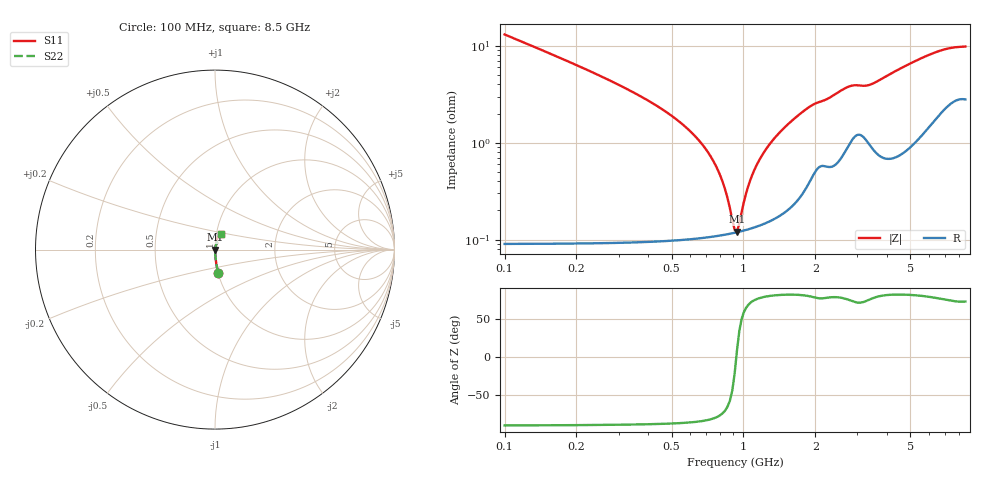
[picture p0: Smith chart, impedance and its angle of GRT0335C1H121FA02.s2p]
!Murata Part Number: GRT0335C1H121FA02
!These Parameters are Measured in Series Mode Connection
!Data Generated on Jun 19, 2026
!  o--ll--o
!Port1  Port2
!  o------o
!Operation Temp=25[degC], DC Bias Voltage=0[V]
!Freq. Start=100[MHz] Stop=9[GHz] 401[Steps]
# Hz S RI R 50
!Freq.(Hz) S11(Real) S11(Imag) S21(Real) S21(Imag) S12(Real) S12(Imag) S22(Real) S22(Imag)
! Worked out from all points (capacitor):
!   401 points, 100 MHz to 8.5 GHz, reference 50 ohm
!   read as one part in series: C = 120 pF near 142 MHz
!   lowest |Z| = 121 mohm at 940 MHz (marker M1)
!   series resonance near 933.6 MHz, so ESL is about 240 pH
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1e8  0.0178 -0.1287  0.9822 0.1287  0.9822 0.1287  0.0178 -0.1287
2.05e8  0.00468 -0.0613  0.9953 0.0613  0.9953 0.0613  0.00468 -0.0613
2.68e8  0.00298 -0.0453  0.997 0.0453  0.997 0.0453  0.00298 -0.0453
5.83e8  0.0012 -0.0139  0.9988 0.0139  0.9988 0.0139  0.0012 -0.0139
7.09e8  0.00112 -0.00796  0.9989 0.00796  0.9989 0.00796  0.00112 -0.00796
8.14e8  0.00113 -0.00393  0.9989 0.00393  0.9989 0.00393  0.00113 -0.00393
8.98e8  0.00116 -0.00111  0.9988 0.00111  0.9988 0.00111  0.00116 -0.00111
9.19e8  0.00118 -0.000451  0.9988 0.000451  0.9988 0.000451  0.00118 -0.000451
9.4e8  0.00119 0.000197  0.9988 -0.000197  0.9988 -0.000197  0.00119 0.000197
9.61e8  0.00121 0.000832  0.9988 -0.000832  0.9988 -0.000832  0.00121 0.000832
1.066e9  0.00131 0.00384  0.9987 -0.00384  0.9987 -0.00384  0.00131 0.00384
1.15e9  0.00141 0.00607  0.9986 -0.00607  0.9986 -0.00607  0.00141 0.00607
1.297e9  0.00165 0.00974  0.9984 -0.00974  0.9984 -0.00974  0.00165 0.00974
1.507e9  0.00216 0.0147  0.9978 -0.0147  0.9978 -0.0147  0.00216 0.0147
1.948e9  0.00505 0.0239  0.9949 -0.0239  0.9949 -0.0239  0.00505 0.0239
2.662e9  0.00921 0.035  0.9908 -0.035  0.9908 -0.035  0.00921 0.035
2.914e9  0.0127 0.0366  0.9873 -0.0366  0.9873 -0.0366  0.0127 0.0366
3.376e9  0.0108 0.0377  0.9892 -0.0377  0.9892 -0.0377  0.0108 0.0377
4.3e9  0.00979 0.053  0.9902 -0.053  0.9902 -0.053  0.00979 0.053
5.707e9  0.018 0.0735  0.982 -0.0735  0.982 -0.0735  0.018 0.0735
7.114e9  0.0304 0.0857  0.9696 -0.0857  0.9696 -0.0857  0.0304 0.0857
8.5e9  0.0354 0.0886  0.9646 -0.0886  0.9646 -0.0886  0.0354 0.0886
